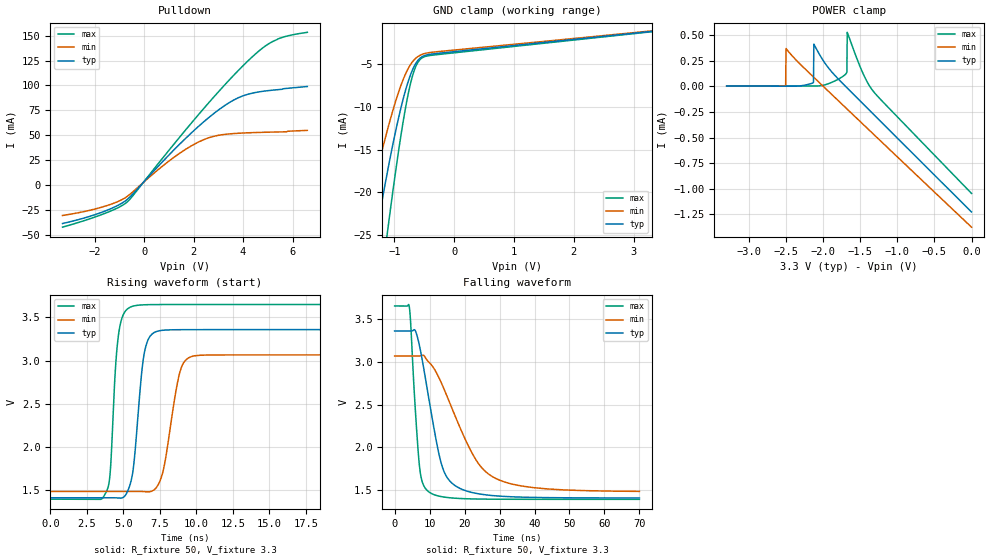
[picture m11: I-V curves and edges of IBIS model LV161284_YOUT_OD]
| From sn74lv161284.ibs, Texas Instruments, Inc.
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[Model]   LV161284_YOUT_OD
Model_type  Open_drain
Enable   Active-Low
Vref =   3.3
Rref =   500
Cref =   50p
Vmeas =   1.4
| variable   typ   min   max
C_comp   4.69pF   4.14pF   5.18pF
| C_pulldown   4.34pF   3.78pF   4.90pF
| C_tri-state   4.69pF   4.14pF   5.18pF
[Temperature Range]   40   100   -40
| Ambient temperature   25   85   -40
[Voltage range]   3.3   3   3.6
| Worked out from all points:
|   slope of the pulldown table from 0 to 0.495 V, typ, clamps not added: 37 ohm
|   rising waveform, R_fixture 50, V_fixture 3.3: 20-80 % time 613ps typ, 892ps min, 444ps max; typ from 1.41 V to 3.36 V
|   falling waveform, R_fixture 50, V_fixture 3.3: 20-80 % time 5.32ns typ, 10.8ns min, 2.04ns max; typ from 3.36 V to 1.41 V
[GND Clamp]
| LV161284_YOUT_OD
|   Voltage   I(typ)   I(min)   I(max)
-3.3V     -128.5mA   -91.9mA    -165.3mA
-1.54V    -35.06mA   -25.15mA   -49.34mA
-1.495V   -33.05mA   -23.72mA   -46.6mA
-1.295V   -24.56mA   -17.67mA   -34.74mA
-1.275V   -23.75mA   -17.09mA   -33.58mA
-1.11V    -17.41mA   -12.58mA   -24.37mA
-920mV    -11.04mA   -8.128mA   -14.75mA
-785mV    -7.438mA   -5.784mA   -9.11mA
-675mV    -5.391mA   -4.592mA   -5.938mA
-560mV    -4.291mA   -3.978mA   -4.444mA
-370mV    -3.863mA   -3.66mA    -4.005mA
3.3V      -1.226mA   -1.168mA   -1.268mA
[POWER Clamp]
| LV161284_YOUT_OD
|   Voltage   I(typ)   I(min)   I(max)
-3.3V     300nA      12.91nA    4.168uA
-2.505V   190.8nA    4.994uA    2.526uA
-2.5V     190.5nA    367uA      2.518uA
-2.13V    36.27uA    89.82uA    1.969uA
-2.125V   410uA      86.36uA    1.972uA
-1.94V    189.5uA    -41.39uA   21.58uA
-1.685V   -10.58uA   -217.2uA   128.7uA
-1.68V    -14.21uA   -220.7uA   137.2uA
-1.675V   -17.83uA   -224.1uA   525uA
-1.475V   -162.4uA   -361.8uA   145uA
-1.33V    -267.1uA   -461.6uA   -43.62uA
-48.03fV  -1.226mA   -1.373mA   -1.045mA
[Pulldown]
| LV161284_YOUT_OD
|   Voltage   I(typ)   I(min)   I(max)
-3.3V     -38.49mA   -30.42mA   -42.13mA
-1.69V    -27.01mA   -21.92mA   -29.3mA
-1.045V   -20.07mA   -16.3mA    -22.51mA
-680mV    -14.27mA   -11.21mA   -16.75mA
810mV     25.23mA    20.41mA    29.02mA
1.84V     50.74mA    38.38mA    60.19mA
2.68V     69.12mA    48.05mA    84.54mA
3.58V     84.76mA    51.67mA    109.1mA
4.215V    91.3mA     52.52mA    125mA
5.08V     94.99mA    53.16mA    142.4mA
5.665V    96.78mA    53.47mA    148.8mA
6.6V      98.93mA    54.94mA    153.3mA
[Ramp]
| LV161284_YOUT_OD
| variable   typ   min   max
dV/dt_r   1.17/6.20E-10   0.95/8.97E-10   1.36/4.52E-10
dV/dt_f   1.18/5.34E-09   0.95/1.08E-08   1.36/2.05E-09
R_load = 50
[Rising Waveform]
| LV161284_YOUT_OD
R_fixture =   50
C_fixture =   0
L_fixture =   0
V_fixture =   3.3
V_fixture_min = 3
V_fixture_max = 3.6
|   Time   V(typ)   V(min)   V(max)
0s        1.409V     1.483V     1.393V
3.865ns   1.409V     1.483V     1.489V
4.1ns     1.409V     1.483V     1.7V
4.71ns    1.406V     1.483V     3.346V
5.81ns    1.96V      1.483V     3.637V
6.725ns   3.253V     1.478V     3.648V
7.685ns   3.351V     1.695V     3.65V
8.95ns    3.358V     2.911V     3.65V
9.925ns   3.359V     3.057V     3.65V
70ns      3.359V     3.066V     3.65V
[Falling Waveform]
| LV161284_YOUT_OD
R_fixture =   50
C_fixture =   0
L_fixture =   0
V_fixture =   3.3
V_fixture_min = 3
V_fixture_max = 3.6
|   Time   V(typ)   V(min)   V(max)
0s        3.359V     3.066V     3.65V
4.18ns    3.359V     3.066V     3.646V
5.855ns   3.367V     3.066V     2.487V
7.085ns   3.192V     3.066V     1.792V
9.69ns    2.593V     2.999V     1.483V
13.75ns   1.759V     2.717V     1.422V
18.67ns   1.521V     2.234V     1.403V
24.47ns   1.455V     1.784V     1.397V
30.84ns   1.429V     1.604V     1.394V
70ns      1.409V     1.486V     1.393V
